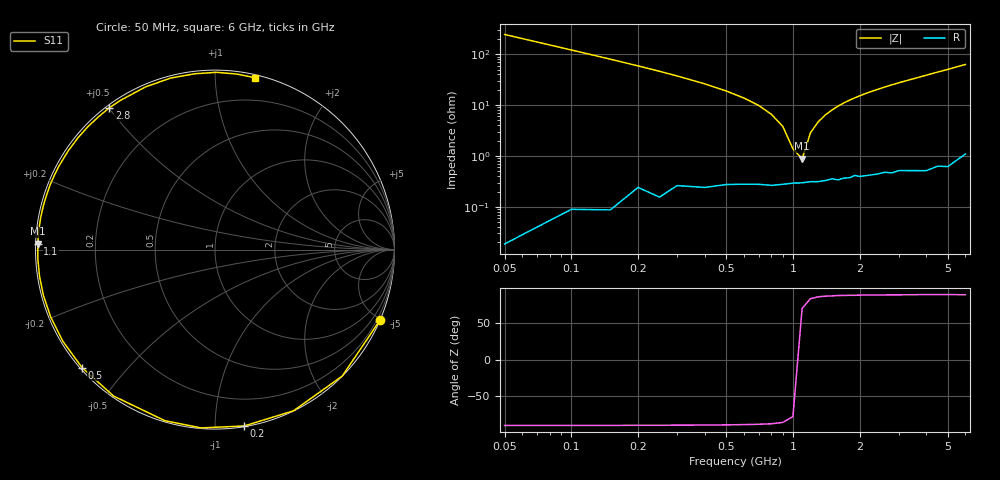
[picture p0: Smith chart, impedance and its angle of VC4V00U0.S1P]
! Infineon Technologies  Discrete & RF Semiconductors
! BBY 56-03
! Si Tuning Diode in SOD323
! VR = 4 V
! S-Parameters:  June  1999
# GHz  S  MA  R  50
!  f  S11
! GHz  MAG  ANG
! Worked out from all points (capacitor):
!   34 points, 50 MHz to 6 GHz, reference 50 ohm
!   read as one part to ground: C = 13 pF near 50 MHz
!   lowest |Z| = 881 mohm at 1.1 GHz (marker M1)
!   series resonance near 1.062 GHz, so ESL is about 1.7 nH
!   S11 on the Smith chart (normalised r, x): 50 MHz: 0.00, -4.89; 200 MHz: 0.00, -1.18; 500 MHz: 0.01, -0.38; 1.1 GHz: 0.01, +0.02; 2.8 GHz: 0.01, +0.50; 6 GHz: 0.02, +1.26
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0.05  1 -23.1
0.1  0.9995 -44.8
0.15  0.999 -64.0
0.2  0.996 -80.6
0.25  0.9967 -94.5
0.3  0.9933 -106.3
0.4  0.9925 -124.7
0.5  0.9904 -138.4
0.6  0.9897 -149.1
0.7  0.9894 -157.7
0.8  0.9896 -165.0
0.9  0.989 -171.3
1  0.9883 -176.9
1.1  0.9882 178.1
1.3  0.9876 169.3
1.6  0.987 158.3
1.8  0.9861 151.9
2  0.9856 146.1
2.2  0.9852 140.7
2.4  0.985 135.8
2.8  0.9852 126.7
3  0.9842 122.5
3.5  0.9857 113.1
4  0.9872 104.4
4.5  0.986 96.5
5  0.9878 89.5
5.5  0.9855 82.8
6  0.9832 77.0
